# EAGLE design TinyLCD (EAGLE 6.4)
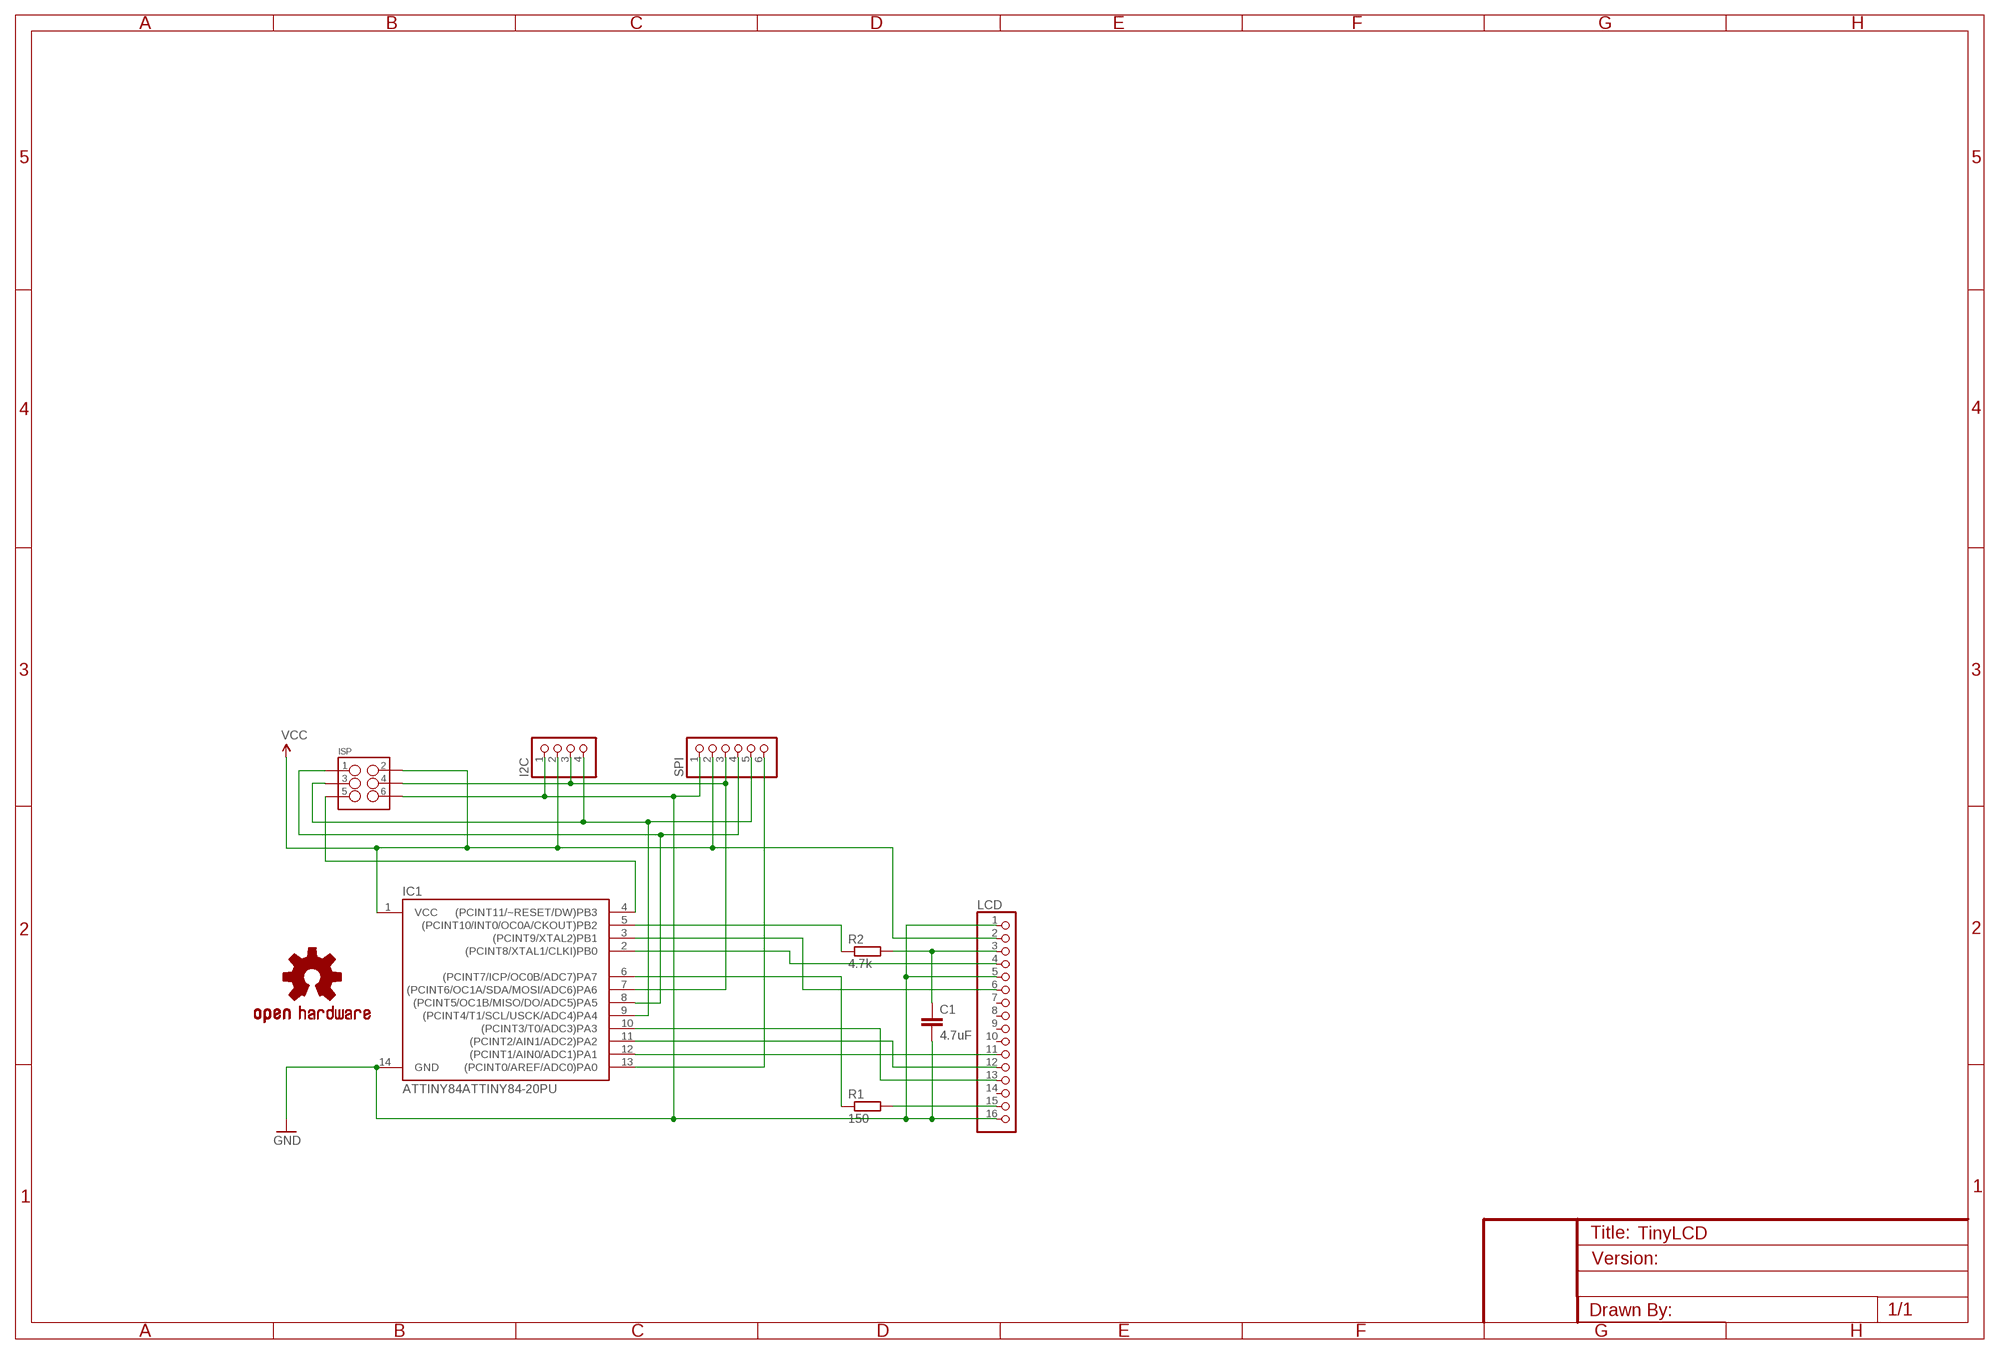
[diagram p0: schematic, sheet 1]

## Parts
C1  4.7uF  C-EU025-030X050  [C025-030X050]
I2C  PINHD-1X4  [1X04]
IC1  ATTINY84ATTINY84-20PU  [DIL14]
ISP  M03X2  [2X3-SHROUDED]
LCD  PINHD-1X16  [1X16]
LOGO1  OSHW-LOGOS  [OSHW-LOGO-S]
R1  150  R-EU_0207/10  [0207/10]
R2  4.7k  R-EU_0207/10  [0207/10]
SPI  PINHD-1X6  [1X06]

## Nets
GND: C1.2 I2C.1 IC1.14(GND) ISP.6 LCD.1 LCD.5 LCD.16 SPI.1
N$1: IC1.2((PCINT8/XTAL1/CLKI)PB0) LCD.4
N$2: IC1.3((PCINT9/XTAL2)PB1) LCD.6
N$3: C1.1 LCD.3 R2.2
N$4: IC1.5((PCINT10/INT0/OC0A/CKOUT)PB2) R2.1
N$5: IC1.4((PCINT11/~RESET/DW)PB3) ISP.5
N$6: I2C.3 IC1.7((PCINT6/OC1A/SDA/MOSI/ADC6)PA6) ISP.4 SPI.3
N$7: IC1.13((PCINT0/AREF/ADC0)PA0) SPI.6
N$8: LCD.15 R1.2
N$9: IC1.6((PCINT7/ICP/OC0B/ADC7)PA7) R1.1
N$10: I2C.4 IC1.9((PCINT4/T1/SCL/USCK/ADC4)PA4) ISP.3 SPI.5
N$11: IC1.8((PCINT5/OC1B/MISO/DO/ADC5)PA5) ISP.1 SPI.4
N$12: IC1.11((PCINT2/AIN1/ADC2)PA2) LCD.12
N$13: IC1.12((PCINT1/AIN0/ADC1)PA1) LCD.11
N$14: IC1.10((PCINT3/T0/ADC3)PA3) LCD.13
VCC: I2C.2 IC1.1(VCC) ISP.2 LCD.2 SPI.2
Unconnected: LCD.7 LCD.8 LCD.9 LCD.10 LCD.14

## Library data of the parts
C1 = rcl:C-EU: CAPACITOR, European symbol
I2C = pinhead:PINHD-1X4: PIN HEADER
IC1 = SparkFun-DigitalIC:ATTINY84: Atmel 14-pin 2/4/8kB flash uC
ISP = SparkFun-Connectors:M03X2: 2x3 .1" header. Shrouded, with keying- CONN-10681 SMT- CONN-11415 Pogo pins- HW-11044; PROD_ID: CONN-10681
LCD = pinhead:PINHD-1X16: PIN HEADER
LOGO1 = SparkFun-Aesthetics:OSHW-LOGO: Open Source Hardware Logo This logo indicates the piece of hardware it is found on incorporates a OSHW license and/or adheres to the definition of open source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
R1 R2 = rcl:R-EU_: RESISTOR, European symbol
SPI = pinhead:PINHD-1X6: PIN HEADER

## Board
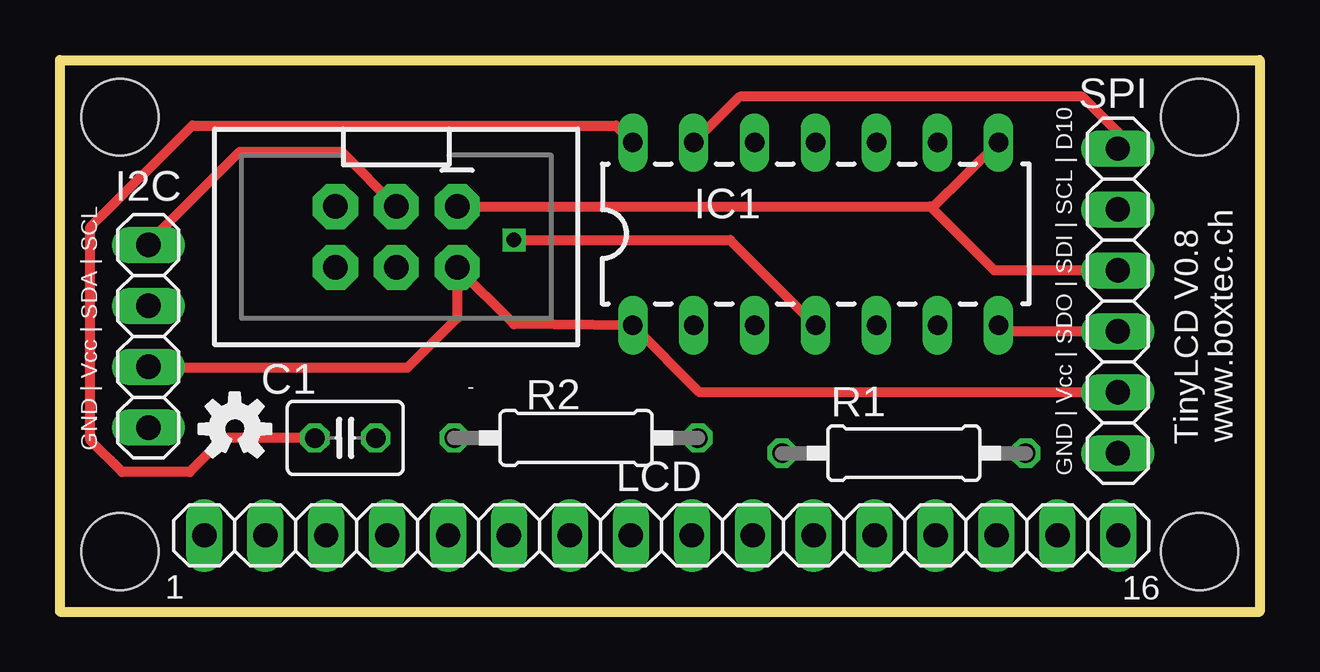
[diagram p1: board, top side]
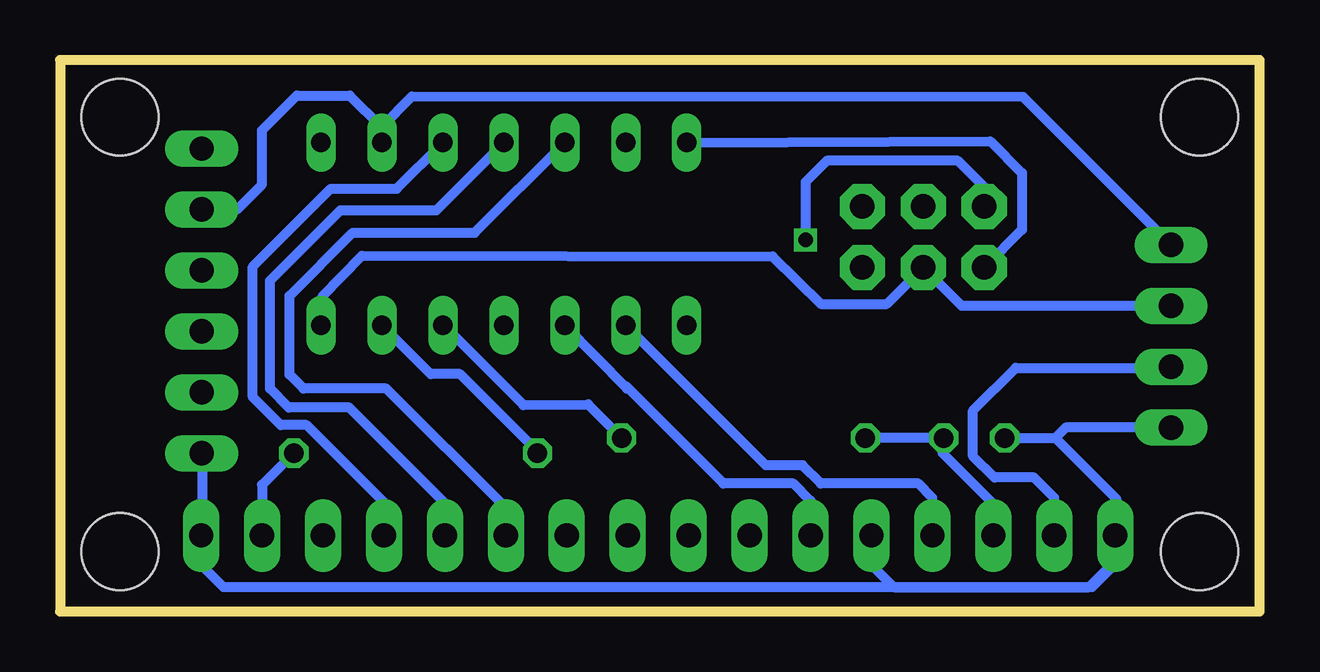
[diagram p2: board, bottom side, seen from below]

Size 50 x 23 mm. Coordinates in mm from the lower left corner, seen from the top.
Outline: 0,0 50,0 50,23 0,23 0,0
Copper layers (1*16): Top 0.0356mm / dielectric 1.5011mm / Bottom 0.0356mm
Design rules "LaenPCBOrder": minimum track width 6mil, minimum drill 13mil, track to track 6mil, track to pad 6mil, pad to pad 6mil, via to via 6mil, smd to smd 6mil, copper to edge 15mil, drill to drill 6mil, minimum pad ring 7mil, minimum via ring 7mil, stop-mask expansion 4mil, vias tented up to drill 0mil, thermal gap 10mil
Holes 3.2 mm at 2.5,2.5 47.5,2.5 47.5,20.62 2.5,20.62

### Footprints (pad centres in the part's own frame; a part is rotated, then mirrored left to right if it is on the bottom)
C025-030X050 = drill 0.813 octagon: 1 -1.27,0; 2 1.27,0
1X04 = drill 1.016 long: 1 -3.81,0; 2 -1.27,0; 3 1.27,0; 4 3.81,0
DIL14 = drill 0.813 long: 1 -8.89,-3.81; 2 -6.35,-3.81; 3 -3.81,-3.81; 4 -1.27,-3.81; 5 1.27,-3.81; 6 3.81,-3.81; 7 6.35,-3.81; 8 6.35,3.81; 9 3.81,3.81; 10 1.27,3.81; 11 -1.27,3.81; 12 -3.81,3.81; 13 -6.35,3.81; 14 -8.89,3.81
2X3-SHROUDED = drill 1.016 pad 1.88 octagon: 1 -1.27,2.54; 2 1.27,2.54; 3 -1.27,0; 4 1.27,0; 5 -1.27,-2.54; 6 1.27,-2.54
1X16 = drill 1.016 long: 1 -19.05,0; 2 -16.51,0; 3 -13.97,0; 4 -11.43,0; 5 -8.89,0; 6 -6.35,0; 7 -3.81,0; 8 -1.27,0; 9 1.27,0; 10 3.81,0; 11 6.35,0; 12 8.89,0; 13 11.43,0; 14 13.97,0; 15 16.51,0; 16 19.05,0
0207/10 = drill 0.813 octagon: 1 -5.08,0; 2 5.08,0
1X06 = drill 1.016 long: 1 -6.35,0; 2 -3.81,0; 3 -1.27,0; 4 1.27,0; 5 3.81,0; 6 6.35,0

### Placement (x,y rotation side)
C1  11.89,7.24 180 top
I2C  3.68,11.48 90 top
IC1  32.77,15.74 0 top
ISP  14.02,15.62 270 top
LCD  25.07,3.17 0 top
LOGO1  7.29,7.62 0 top
R1  35.18,6.6 0 top
R2  21.51,7.24 180 top
SPI  44.09,12.95 90 top

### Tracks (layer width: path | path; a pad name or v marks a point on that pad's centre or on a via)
GND
  Top 0.406: C1.2 6.83,7.24 5.41,5.82 2.59,5.82 1.27,7.14 1.27,16.03 5.51,20.27 23.16,20.27 IC1.14
  Bottom 0.406: 6.02,4.75 LCD.1 5.97,3.13 | 6.02,4.75 8.51,7.24 | I2C.1 8.08,7.67 8.51,7.24 | IC1.14 11.22,19.61 9.91,18.29 9.91,15.92 ISP.6 | LCD.5 16.18,1.95 15.24,1.02 7.11,1.02 5.97,2.16 | 5.97,2.16 5.97,3.13 | C1.2 8.51,7.24 | 6.02,4.75 5.97,4.7 5.97,3.13 | 5.97,2.16 5.97,2.03 6.99,1.02 43.18,1.02 44.2,2.03 44.2,3.1 LCD.16 44.04,3.25 44.04,6.55 SPI.1
N$1
  Bottom 0.406: LCD.4 13.64,4.75 14.22,5.33 18.29,5.33 19.05,6.1 20.58,6.1 IC1.2
N$2
  Bottom 0.406: LCD.6 18.72,4.62 19.43,5.33 22.35,5.33 26.42,9.4 26.37,9.3 IC1.3
N$3
  Bottom 0.406: LCD.3 11.1,4.49 13.21,6.6 13.21,7.19 C1.1 R2.2
N$4
  Bottom 0.406: IC1.5 34.03,11.96 30.68,8.61 27.99,8.64 R2.1
N$5  (via drill 0.6)
  Top 0.406: v18.92,15.49 27.94,15.49 IC1.4
  Bottom 0.406: ISP.5 11.48,17.7 12.57,18.8 18.03,18.8 18.92,17.91 v18.92,15.49
N$6
  Top 0.406: SPI.3 39.37,11.68 IC1.7
  Bottom 0.406: IC1.7 39.06,13.13 37.41,14.83 20.3,14.81 18.29,12.83 15.54,12.83 ISP.4 12.41,12.75 I2C.3
N$7
  Top 0.406: SPI.6 44.09,19.99 42.62,21.46 28.32,21.46 IC1.13
N$8
  Bottom 0.406: R1.2 41.58,5.28 LCD.15
N$9
  Bottom 0.406: R1.1 30.09,6.68 33.33,9.91 34.55,9.91 IC1.6
N$10
  Top 0.406: I2C.4 3.68,15.37 7.49,19.18 11.73,19.18 ISP.3
  Bottom 0.406: IC1.9 36.6,20.19 | 36.6,20.19 35.33,21.49 9.86,21.46 I2C.4 | SPI.5 42.62,16.76 41.58,17.8 41.58,20.07 40.13,21.51 37.92,21.51 36.6,20.19
N$11
  Top 0.406: ISP.1 36.27,16.89 | 36.27,16.89 36.4,16.89 IC1.8 | SPI.4 38.94,14.22 36.27,16.89
N$12
  Bottom 0.406: LCD.12 33.96,4.52 37.95,8.51 40.46,8.51 41.25,9.3 41.25,13.79 38.3,16.74 34.31,16.74 IC1.11
N$13
  Bottom 0.406: LCD.11 31.42,4.31 36.4,9.3 39.85,9.3 40.44,9.88 40.44,13.16 37.8,15.8 32.71,15.8 IC1.12
N$14
  Bottom 0.406: LCD.13 36.5,4.54 39.73,7.77 40.79,7.77 41.96,8.94 41.96,14.38 38.71,17.63 35.96,17.63 IC1.10
VCC
  Top 0.406: I2C.2 3.73,10.16 14.48,10.16 16.56,12.24 ISP.2 18.92,11.98 IC1.1 26.67,9.14 SPI.2
  Bottom 0.406: LCD.2 8.56,4.75 9.4,5.59 11.05,5.59 11.94,6.48 11.94,8.38 10.16,10.16 3.73,10.16 I2C.2

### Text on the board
tNames: GND | Vcc | SDA | SCL | TinyLCD V0.8 | www.boxtec.ch | GND | Vcc | SDO | SDI | SCL | D10 | 1 | 16

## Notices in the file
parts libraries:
SparkFun-Aesthetics: Licensing: CC v3.0 Share-Alike You are welcome to use this library for commercial purposes.
